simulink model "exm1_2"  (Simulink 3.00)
settings: Solver=ode45  StartTime=0.0  StopTime=5  MaxStep=1e-3  RelTol=1e-3
libraries: simulink3 x1

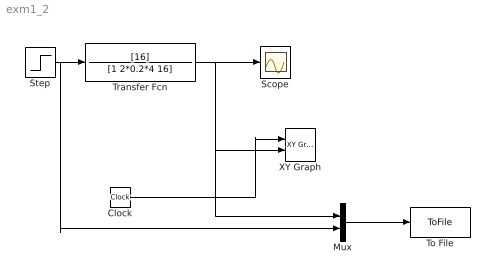
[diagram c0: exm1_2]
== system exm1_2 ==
  Clock : Clock
  Mux : Mux  Inputs=2
  Scope : Scope
  Step : Step  Time=0  Before=0  After=1  SampleTime=0
  To File : ToFile  Filename=s.mat  MatrixName=st  SampleTime=-1
  Transfer Fcn : TransferFcn  Numerator=[16]  Denominator=[1 2*0.2*4 16]
  XY Graph : simulink3/Sinks/XY Graph  xmin=0  xmax=5  ymin=0  ymax=2  st=-1
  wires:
  Clock/1 -> XY Graph/1
  Transfer Fcn/1 -> Scope/1, XY Graph/2, Mux/1
  Step/1 -> Transfer Fcn/1, Mux/2
  Mux/1 -> To File/1
